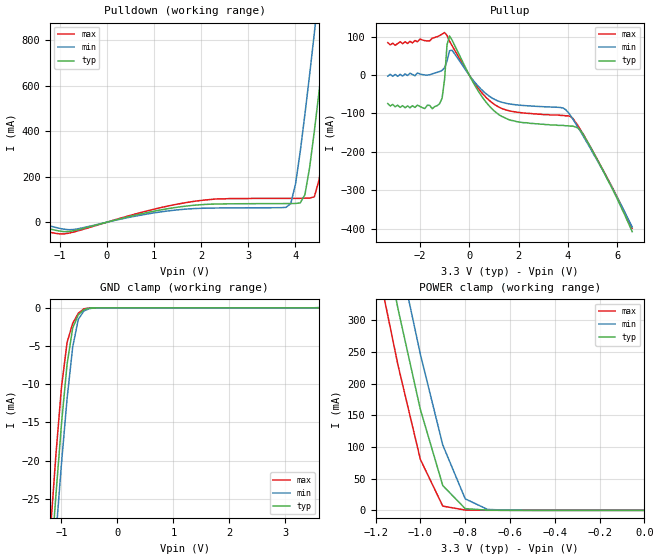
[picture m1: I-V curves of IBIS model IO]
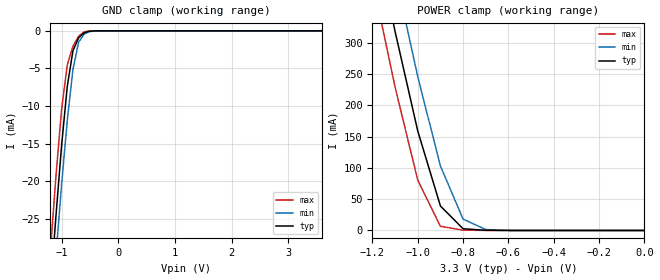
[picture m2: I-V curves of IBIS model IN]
[IBIS Ver]   1.1
[File name]   63919tq.ibs
[File Rev]   1.0
[Date]   September 27, 1999
[Source]   This file originated at Motorola Fast SRAM.
[Notes]
1. This I/O model good for MCM63919 512Kx18 BurstRAM "F" and "P" versions
[Disclaimer]   Data is for modeling purposes only and is not guaranteed
[Component]   512Kx18 8Mb BurstRAM
[Manufacturer] Motorola
[Package]
|  RLC Data is subject to change after further study of package
|		typ		min		max
R_pkg		200m		150m		250m
L_pkg		5.5nH		4nH		7nH
C_pkg		2pF		1.5pF		2.5pF
[Pin]		signal_name	model_name	R_pin		L_pin		C_pin
1		NC		NC		NA		NA		NA
2		NC		NC		NA		NA		NA
3		NC		NC		NA		NA		NA
4		VDDQ		POWER		NA		NA		NA
5		VSS		GND		NA		NA		NA
6		NC		NC		NA		NA		NA
7		NC		NC		NA		NA		NA
8		DQb		IO		NA		NA		NA
9		DQb		IO		NA		NA		NA
10		VSS		GND		NA		NA		NA
11		VDDQ		POWER		NA		NA		NA
12		DQb		IO		NA		NA		NA
13		DQb		IO		NA		NA		NA
14		NC		NC		NA		NA		NA
15		VDD		POWER		NA		NA		NA
16		NC		NC		NA		NA		NA
17		VSS		GND		NA		NA		NA
18		DQb		IO		NA		NA		NA
19		DQb	 	IO		NA		NA		NA
20		VDDQ		POWER		NA		NA		NA
21		VSS		GND		NA		NA		NA
22		DQb		IO		NA		NA		NA
23		DQb		IO		NA		NA		NA
24		DQb		IO		NA		NA		NA
25		NC		NC		NA		NA		NA
26		VSS		GND		NA		NA		NA
27		VDDQ		POWER		NA		NA		NA
28		NC		NC		NA		NA		NA
29		NC		NC		NA		NA		NA
30		NC		NC		NA		NA		NA
31		LBO#		IN		NA		NA		NA
32		SA		IN		NA		NA		NA
33		SA		IN		NA		NA		NA
34		SA		IN		NA		NA		NA
35		SA		IN		NA		NA		NA
36		SA1		IN		NA		NA		NA
37		SA0		IN		NA		NA		NA
38		NC		NC		NA		NA		NA
39		NC		NC		NA		NA		NA
40		VSS		GND		NA		NA		NA
41		VDD		POWER		NA		NA		NA
42		NC		NC		NA		NA		NA
43		SA		IN		NA		NA		NA
44		SA		IN		NA		NA		NA
45		SA		IN		NA		NA		NA
46		SA		IN		NA		NA		NA
47		SA		IN		NA		NA		NA
48		SA		IN		NA		NA		NA
49		SA		IN		NA		NA		NA
50		SA		IN		NA		NA		NA
51		NC		NC		NA		NA		NA
52		NC		NC		NA		NA		NA
53		NC		NC		NA		NA		NA
54		VDDQ		POWER		NA		NA		NA
55		VSS		GND		NA		NA		NA
56		NC		NC		NA		NA		NA
57		NC		NC		NA		NA		NA
58		DQa		IO		NA		NA		NA
59		DQa		IO		NA		NA		NA
60		VSS		GND		NA		NA		NA
61		VDDQ		POWER		NA		NA		NA
62		DQa		IO		NA		NA		NA
63		DQa		IO		NA		NA		NA
64		ZZ		IN		NA		NA		NA
65		VDD		POWER		NA		NA		NA
66		NC		NC		NA		NA		NA
67		VSS		GND		NA		NA		NA
68		DQa		IO		NA		NA		NA
69		DQa		IO		NA		NA		NA
70		VDDQ		POWER		NA		NA		NA
71		VSS		GND		NA		NA		NA
72		DQa		IO		NA		NA		NA
73		DQa		IO		NA		NA		NA
74		DQa		IO		NA		NA		NA
75		NC		NC		NA		NA		NA
76		VSS		GND		NA		NA		NA
77		VDDQ		POWER		NA		NA		NA
78		NC		NC		NA		NA		NA
79		NC		NC		NA		NA		NA
80		SA		IN		NA		NA		NA
81		SA		IN		NA		NA		NA
82		SA		IN		NA		NA		NA
83		ADV#		IN		NA		NA		NA
84		ADSP#		IN		NA		NA		NA
85		ADSC#		IN		NA		NA		NA
86		G#		IN		NA		NA		NA
87		SW#		IN		NA		NA		NA
88		SGW#		IN		NA		NA		NA
89		K		IN		NA		NA		NA
90		VSS		GND		NA		NA		NA
91		VDD		POWER		NA		NA		NA
92		SE3#		IN		NA		NA		NA
93		SBa#		IN		NA		NA		NA
94		SBb#		IN		NA		NA		NA
95		NC		NC		NA		NA		NA
96		NC		NC		NA		NA		NA
97		SE2		IN		NA		NA		NA
98		SE1#		IN		NA		NA		NA
99		SA		IN		NA		NA		NA
100		SA		IN		NA		NA		NA
| Models and submodels in the file (2): IO (I/O), IN (Input)
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| BI-DIRECTIONAL I/O MODEL
[Model]   IO
Model_type  I/O
Polarity   Non-Inverting
Enable   Active-Low
|signals  DQa, DQb
|Variable   typ   min   max
C_comp   3pF   NA   5pF
|Variable   typ   min   max
[Voltage range]   3.3   3.1   3.5
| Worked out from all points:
|   slope of the pulldown table from 0 to 0.495 V, typ, clamps not added: 19.1 ohm
|   slope of the pullup table from 0 to 0.495 V, typ, clamps not added: 9.13 ohm
|   GND clamp passes 1 mA (typ) near -0.70 V on its own axis
|   POWER clamp passes 1 mA (typ) near -0.73 V on its own axis
|Temp used   50C   100C   0C
|Variable   typ   min   max
|NOTE: All V/I tables should have at least 3 entries.
|   0.0 volts, 2*supply_voltage and -supply_voltage
[Pulldown]
|Volt	Typical		Minimum		Maximum
-3.3V     -1.51mA    -548uA     -907uA
-900mV    -41.5mA    -31mA      -51.4mA
1.7V      71.5mA     58mA       87.1mA
3.8V      82.1mA     65.4mA     105mA
3.9V      82.2mA     82.2mA     105mA
4.1V      85mA       310mA      105mA
4.2V      121mA      475mA      106mA
4.4V      401mA      832mA      112mA
4.6V      756mA      1.2A       335mA
4.7V      941mA      1.39A      507mA
4.9V      1.32A      1.77A      874mA
6.6V      4.63A      5.09A      4.19A
[Pullup]
|Volt	Typical		Minimum		Maximum
-3.3V     -74.2mA    -2.51mA    84.6mA
-1.5V     -87.6mA    3.24mA     96.2mA
-1.2V     -74.4mA    9.33mA     103mA
-1.1V     -60.1mA    12.4mA     107mA
-1V       -10.8mA    19.2mA     111mA
-900mV    79.6mA     36.6mA     103mA
-800mV    102mA      63.5mA     88.3mA
300mV     -34.8mA    -24.4mA    -28.9mA
1.1V      -98.2mA    -65.6mA    -79.8mA
3.9V      -132mA     -89.7mA    -106mA
4.6V      -153mA     -157mA     -152mA
6.6V      -408mA     -396mA     -399mA
[GND_clamp]
|Volt	Typical		Minimum		Maximum
-3.6V     -305mA     -302mA     -308mA
-1.2V     -34.7mA    -39.9mA    -29.5mA
-1.1V     -24.6mA    -29.9mA    -19.3mA
-1V       -15.2mA    -20.4mA    -10.4mA
-900mV    -7.38mA    -11.9mA    -4.53mA
-800mV    -2.65mA    -5.14mA    -2.04mA
-700mV    -921uA     -1.51mA    -704uA
-600mV    -243uA     -407uA     -128uA
-500mV    -39.8uA    -94.1uA    -10.8uA
-300mV    -249nA     -1.62uA    -20nA
3.6V      77.9nA     36.8uA     57.2pA
[POWER_clamp]
|Volt	Typical		Minimum		Maximum
-3.7V     5.32A      5.4A       5.24A
-1.2V     492mA      586mA      401mA
-1.1V     318mA      411mA      229mA
-1V       159mA      246mA      80.3mA
-900mV    39.1mA     103mA      6.66mA
-800mV    2.74mA     18.2mA     534uA
-700mV    295uA      1.44mA     94.5uA
-600mV    54.3uA     187uA      11.9uA
0V        86.9pA     1nA        50.2pA
[Ramp]
|Variable   typ   min	max
dV/dt_r  1.602/0.532n		NA	NA
dV/dt_f  1.406/0.435n		NA	NA
| STANDARD INPUT MODEL
[Model]   IN
Model_type  Input
Polarity   Non-Inverting
|signals  ADSC#, ADSP#, ADV#, G#, K, SA, SAx, SBx#,
|   SE1#, SE2, SE3#, SGW#, SW#, LBO#, ZZ
|Variable   typ   min   max
C_comp   2pF   NA   4pF
|Variable   typ   min   max
[Voltage range]   3.3   3.1   3.5
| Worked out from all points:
|   GND clamp passes 1 mA (typ) near -0.70 V on its own axis
|   POWER clamp passes 1 mA (typ) near -0.73 V on its own axis
|Temp used   50C   100C   0C
[GND_clamp]
|Volt	Typical		Minimum		Maximum
-3.6V     -305mA     -302mA     -308mA
-1.2V     -34.7mA    -39.9mA    -29.5mA
-1.1V     -24.6mA    -29.9mA    -19.3mA
-1V       -15.2mA    -20.4mA    -10.4mA
-900mV    -7.38mA    -11.9mA    -4.53mA
-800mV    -2.65mA    -5.14mA    -2.04mA
-700mV    -921uA     -1.51mA    -704uA
-600mV    -243uA     -407uA     -128uA
-500mV    -39.8uA    -94.1uA    -10.8uA
-300mV    -249nA     -1.62uA    -20nA
3.6V      77.9nA     36.8uA     57.2pA
[POWER_clamp]
|Volt	Typical		Minimum		Maximum
-3.7V     5.32A      5.4A       5.24A
-1.2V     492mA      586mA      401mA
-1.1V     318mA      411mA      229mA
-1V       159mA      246mA      80.3mA
-900mV    39.1mA     103mA      6.66mA
-800mV    2.74mA     18.2mA     534uA
-700mV    295uA      1.44mA     94.5uA
-600mV    54.3uA     187uA      11.9uA
0V        86.9pA     1nA        50.2pA
